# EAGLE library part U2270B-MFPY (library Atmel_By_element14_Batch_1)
Read/Write Base Station
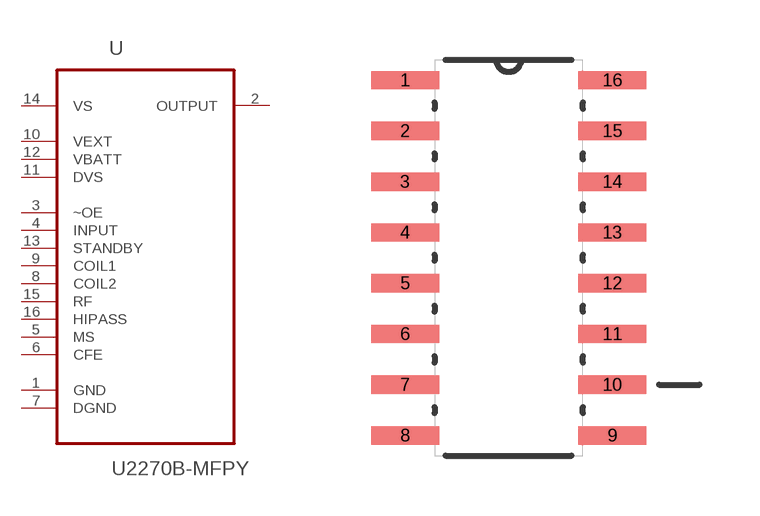
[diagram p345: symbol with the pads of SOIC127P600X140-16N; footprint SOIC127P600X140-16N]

Designator prefix U

## U2270B-MFPY (MPN: U2270B-MFPY; OC_FARNELL: 1095806; OC_NEWARK: 93K1097; PACKAGE: SOIC-16; SUPPLIER: ATMEL)  [SOIC127P600X140-16N]
1  GND  pas
2  OUTPUT  out
3  ~OE  in
4  INPUT  in
5  MS
6  CFE  in
7  DGND  pas
8  COIL2  pas
9  COIL1  pas
10  VEXT  pwr
11  DVS  pwr
12  VBATT  pwr
13  STANDBY  in
14  VS  pwr
15  RF  in
16  HIPASS  in

## Footprint SOIC127P600X140-16N (pad centres in mm)
smd 1.702 x 0.457: 1 -2.591,4.445; 2 -2.591,3.175; 3 -2.591,1.905; 4 -2.591,0.635; 5 -2.591,-0.635; 6 -2.591,-1.905; 7 -2.591,-3.175; 8 -2.591,-4.445; 9 2.591,-4.445; 10 2.591,-3.175; 11 2.591,-1.905; 12 2.591,-0.635; 13 2.591,0.635; 14 2.591,1.905; 15 2.591,3.175; 16 2.591,4.445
